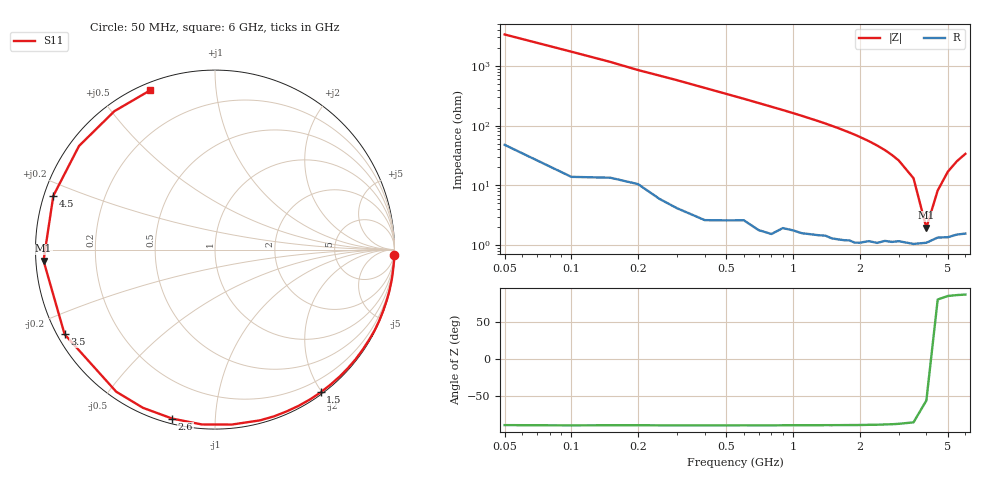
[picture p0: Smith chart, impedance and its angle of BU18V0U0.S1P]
! Infineon Technologies  Discrete & RF Semiconductors
! BB 833
! Si Tuning Diode in SOD323
! VR = 18 V
! S-Parameters:  June  1999
# GHz  S  MA  R  50
!  f  S11
! GHz  MAG  ANG
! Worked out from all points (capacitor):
!   34 points, 50 MHz to 6 GHz, reference 50 ohm
!   read as one part to ground: C = 916 fF near 50 MHz
!   lowest |Z| = 1.95 ohm at 4 GHz (marker M1)
!   series resonance near 4.083 GHz, so ESL is about 1.7 nH
!   S11 on the Smith chart (normalised r, x): 50 MHz: 1, -67; 1.5 GHz: 0.03, -1.98; 2.6 GHz: 0.02, -0.78; 3.5 GHz: 0.02, -0.26; 4.5 GHz: 0.03, +0.16; 6 GHz: 0.03, +0.67
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0.05  0.9996 -1.7
0.25  0.9988 -8.3
0.4  0.9986 -13.3
0.5  0.9978 -16.7
0.6  0.9968 -20.1
0.7  0.997 -23.6
0.8  0.9967 -27.1
1  0.9939 -34.2
1.1  0.9934 -37.9
1.3  0.9913 -45.5
1.4  0.99 -49.4
1.5  0.9896 -53.5
1.6  0.9885 -57.6
1.7  0.9873 -61.9
1.8  0.9859 -66.2
1.9  0.9855 -70.6
2  0.9839 -75.2
2.2  0.9792 -84.5
2.4  0.977 -94.3
2.6  0.9712 -104.2
2.8  0.9686 -114.5
3  0.9642 -124.8
3.5  0.9617 -150.6
4  0.9573 -176.3
4.5  0.9493 161.6
5  0.9526 142.7
5.5  0.9535 126.0
6  0.9581 112.1
